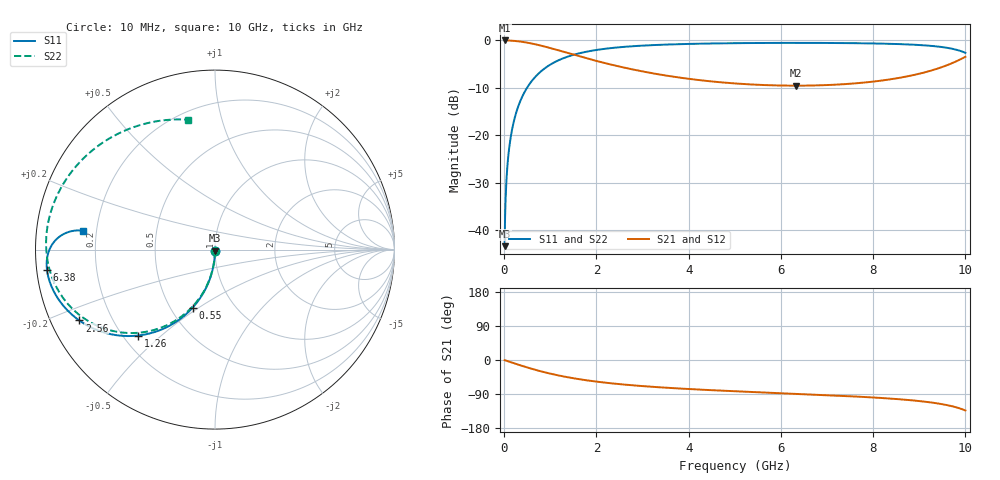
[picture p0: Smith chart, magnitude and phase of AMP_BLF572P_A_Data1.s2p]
! Created Mon Jul 19 16:51:17 2010
# ghz S ma R 50
! 2 Port Network Data from SP1.SP block
! freq  magS11  angS11  magS21  angS21  magS12  angS12  magS22  angS22
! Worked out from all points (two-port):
!   1000 points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, 10 MHz to 10 GHz, reference 50 ohm
!   highest |S21| = 0.00 dB at 10 MHz (marker M1); lowest = -9.5 dB at 6.33 GHz (marker M2)
!   |S21| within 3 dB of the highest: start of sweep to 1.508 GHz
!   lowest |S11| = -43.4 dB at 10 MHz (marker M3), VSWR 1.01, Z = 50 - j0.673 ohm
!   |S11| at or under -10 dB: start of sweep to 496.2 MHz
!   |S22| runs from -43.4 to -0.5 dB; largest |S21 - S12| = 0
!   S11 on the Smith chart (normalised r, x): 10 MHz: 1.00, -0.01; 550 MHz: 0.64, -0.47; 1.26 GHz: 0.26, -0.42; 2.56 GHz: 0.08, -0.24; 6.38 GHz: 0.03, -0.06; 10 GHz: 0.15, +0.07
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0.01  0.006728 -90.4  1 -0.4  1 -0.4  0.006728 -90.4
0.07  0.04704 -92.8  0.9989 -2.9  0.9989 -2.9  0.04704 -92.9
0.09  0.06044 -93.6  0.9982 -3.7  0.9982 -3.7  0.06044 -93.7
0.12  0.08047 -94.8  0.9968 -4.9  0.9968 -4.9  0.08047 -95.0
0.17  0.1136 -96.8  0.9935 -6.9  0.9935 -6.9  0.1136 -97.0
0.24  0.1594 -99.5  0.9872 -9.7  0.9872 -9.7  0.1594 -99.9
0.32  0.2104 -102.6  0.9776 -12.8  0.9776 -12.8  0.2104 -103.1
0.55  0.3465 -111.1  0.938 -21.5  0.938 -21.5  0.3465 -111.9
0.86  0.499 -121.2  0.8666 -31.8  0.8666 -31.8  0.499 -122.5
1.26  0.6423 -131.8  0.7664 -42.8  0.7664 -42.8  0.6423 -133.7
1.68  0.7419 -140.4  0.6705 -51.6  0.6705 -51.6  0.7419 -142.9
2.56  0.8528 -152.4  0.5222 -64.4  0.5222 -64.4  0.8528 -156.3
3.34  0.8982 -159.2  0.4396 -71.8  0.4396 -71.8  0.8981 -164.4
5.01  0.9361 -168.2  0.3515 -82.5  0.3515 -82.5  0.9361 -176.8
6.33  0.9428 -173.0  0.3332 -89.2  0.3332 -89.2  0.9427 174.6
6.38  0.9428 -173.2  0.3332 -89.5  0.3332 -89.5  0.9427 174.3
6.67  0.9424 -174.2  0.3344 -91.0  0.3344 -91.0  0.9423 172.3
8.34  0.9222 180.0  0.3866 -101.5  0.3866 -101.5  0.922 157.0
8.94  0.8988 177.3  0.4382 -107.6  0.4382 -107.6  0.8985 147.6
9.38  0.865 175.0  0.5015 -114.2  0.5015 -114.2  0.8647 136.6
9.71  0.8178 173.0  0.5753 -122.0  0.5753 -122.0  0.8173 123.1
10  0.7404 171.9  0.6718 -133.2  0.6718 -133.2  0.7398 101.9
